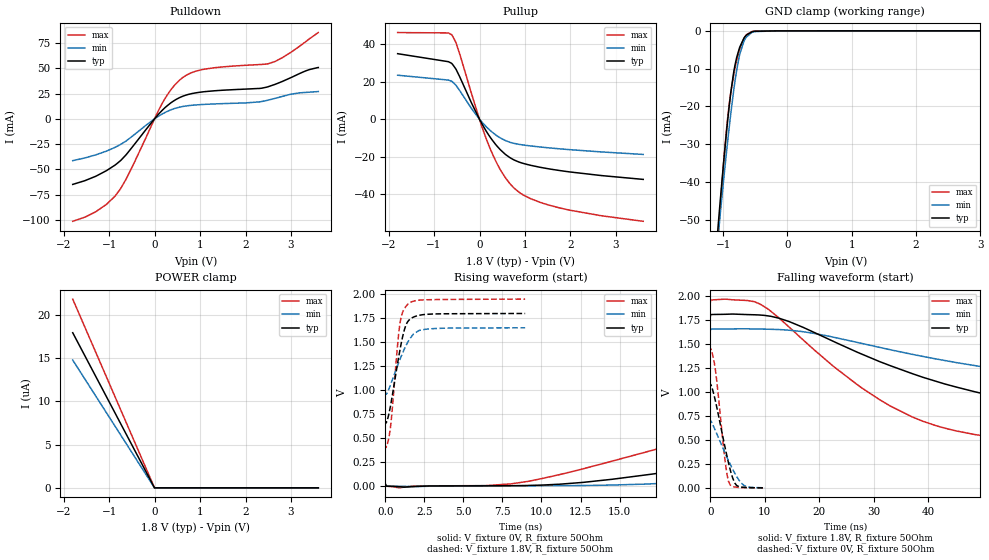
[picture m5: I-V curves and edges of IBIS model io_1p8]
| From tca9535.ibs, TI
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|   io_1p8 Model
[Model]   io_1p8
Model_type   I/O
Polarity   Non-Inverting
Enable   Active-Low
Vinl = 0.54
Vinh = 1.26
Vmeas = 0.9
Vref = 0
Cref = 100pF
Rref = 70
|   typ   min   max
C_comp   2.162e-12   2.013e-12   2.364e-12
[Model spec]
|subparameter
Vinl   0.54   0.495   0.585
Vinh   1.26   1.155   1.365
| Where nom  PVT is Nominal Process, 1.8V, 27C
|   Fast PVT is Strong Process,  1.95V, -40C
|   Slow PVT is Weak Process,   1.65V, 100C
[Voltage Range]   1.8   1.65   1.95
|Junction Temperature
[Temperature Range]   27   100   -40
[Pullup Reference]   1.8   1.65   1.95
[Pulldown Reference]   0   0   0
[Power Clamp Reference]   1.8   1.65   1.95
[GND Clamp Reference]   0   0   0
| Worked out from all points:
|   slope of the pulldown table from 0 to 0.27 V, typ, clamps not added: 21.4 ohm
|   slope of the pullup table from 0 to 0.27 V, typ, clamps not added: 25.1 ohm
|   GND clamp passes 1 mA (typ) near -0.63 V on its own axis
|   falling waveform, V_fixture 1.8V, R_fixture 50Ohm: 20-80 % time 38.2ns typ, 49.8ns min, 23.3ns max; typ from 1.8 V to 0.655 V
|   rising waveform, V_fixture 0V, R_fixture 50Ohm: 20-80 % time 41.8ns typ, 53.4ns min, 26.9ns max; typ from 0 V to 1.07 V
|   rising waveform, V_fixture 1.8V, R_fixture 50Ohm: 20-80 % time 743ps typ, 1.06ns min, 499ps max; typ from 0.653 V to 1.8 V
|   falling waveform, V_fixture 0V, R_fixture 50Ohm: 20-80 % time 2.43ns typ, 3.36ns min, 1.61ns max; typ from 1.07 V to 0.003 V
[Pulldown]
|   Voltage   I(typ)   I(min)   I(max)
-1.8V     -64.95mA   -41.41mA   -101.5mA
-1.288V   -56.76mA   -35.59mA   -91.87mA
-847.9mV  -45.06mA   -27.75mA   -75.37mA
-608.7mV  -34.62mA   -21.35mA   -58.12mA
203.1mV   10.02mA    5.717mA    18.16mA
430.8mV   18.11mA    10.12mA    32.89mA
623.9mV   22.5mA     12.3mA     41.06mA
1.113V    27.02mA    14.39mA    49.37mA
2.317V    30.18mA    16.88mA    53.84mA
2.648V    34.17mA    20.3mA     56.83mA
3.011V    41.15mA    24.57mA    66.34mA
3.6V      50.92mA    27.07mA    85.51mA
[GND Clamp]
|   Voltage   I(typ)   I(min)   I(max)
-1.8V     -224.5mA   -202.8mA   -264.1mA
-1.158V   -68.45mA   -69.08mA   -74.77mA
-1.066V   -49.01mA   -52.08mA   -51.39mA
-1.037V   -43.23mA   -46.97mA   -44.54mA
-990.8mV  -34.41mA   -39.08mA   -34.34mA
-932.3mV  -24.09mA   -29.56mA   -23.33mA
-883.8mV  -16.69mA   -22.24mA   -16.6mA
-837mV    -11.05mA   -15.87mA   -11.74mA
-740.7mV  -4.259mA   -6.106mA   -4.697mA
-665.1mV  -1.66mA    -2.341mA   -1.627mA
-554mV    -267.7uA   -441.4uA   -194.2uA
3.6V      0A         0A         0A
[Pullup]
|   Voltage   I(typ)   I(min)   I(max)
-1.8V     35.04mA    23.52mA    46.35mA
-684mV    30.77mA    20.92mA    46.17mA
-598.8mV  29.53mA    20.05mA    44.75mA
-509.7mV  26.38mA    17.85mA    40.37mA
1.8mV     -167.6uA   -102.1uA   -284.1uA
245.5mV   -10.05mA   -6.293mA   -16.47mA
391.2mV   -14.6mA    -9.037mA   -24.07mA
557.5mV   -18.61mA   -11.32mA   -30.95mA
861.8mV   -22.91mA   -13.45mA   -38.99mA
1.328V    -25.75mA   -14.89mA   -44.5mA
1.76V     -27.5mA    -15.88mA   -47.51mA
3.6V      -32.24mA   -18.88mA   -54.68mA
[POWER Clamp]
|   Voltage   I(typ)   I(min)   I(max)
-1.8V     17.95uA    14.79uA    21.84uA
-54.3mV   524.5nA    435.2nA    636.3nA
-2.1mV    0A         0A         0A
3.6V      0A         0A         0A
[Ramp]
R_load = 50
|   typ   min   max
dV/dt_r   0.641354/4.16014e-08   0.410832/5.32308e-08   0.866703/2.69125e-08
dV/dt_f   0.686979/3.8094e-08   0.415892/4.96413e-08   0.930695/2.32883e-08
[Falling Waveform]
V_fixture = 1.8V
V_fixture_min = 1.65V
V_fixture_max = 1.95V
R_fixture = 50Ohm
|   Time   V(typ)   V(min)   V(max)
0s        1.8V       1.65V      1.95V
9.173ns   1.798V     1.652V     1.912V
14.52ns   1.73V      1.64V      1.671V
23.09ns   1.512V     1.562V     1.244V
32.88ns   1.276V     1.44V      859.9mV
41.37ns   1.112V     1.343V     650.7mV
52.57ns   950.6mV    1.239V     523.8mV
69.05ns   808.3mV    1.131V     451.8mV
93.24ns   717.1mV    1.041V     416.3mV
200ns     655mV      956.8mV    398.8mV
[Rising Waveform]
V_fixture = 0V
V_fixture_min = 0V
V_fixture_max = 0V
R_fixture = 50Ohm
|   Time   V(typ)   V(min)   V(max)
0s        239.1uV    261.6uV    197.6uV
9.173ns   3.748mV    137.6uV    47.16mV
14.52ns   67.89mV    7.953mV    257mV
25.7ns    319.2mV    105.7mV    717.1mV
36.91ns   542.2mV    235.5mV    1.049V
45.22ns   671.2mV    319.9mV    1.204V
56.57ns   802.6mV    413.4mV    1.317V
77.09ns   942.4mV    529.8mV    1.396V
104ns     1.02V      612.3mV    1.429V
200ns     1.069V     685mV      1.445V
[Rising Waveform]
V_fixture = 1.8V
V_fixture_min = 1.65V
V_fixture_max = 1.95V
R_fixture = 50Ohm
|   Time   V(typ)   V(min)   V(max)
0s        653mV      952.8mV    398.6mV
176.2ps   716.7mV    990.7mV    466.6mV
341ps     845mV      1.059V     631.2mV
775ps     1.27V      1.251V     1.457V
931.8ps   1.415V     1.317V     1.69V
1.108ns   1.557V     1.387V     1.811V
1.399ns   1.704V     1.487V     1.888V
1.805ns   1.76V      1.585V     1.926V
2.559ns   1.788V     1.633V     1.941V
8.953ns   1.798V     1.648V     1.948V
[Falling Waveform]
V_fixture = 0V
V_fixture_min = 0V
V_fixture_max = 0V
R_fixture = 50Ohm
|   Time   V(typ)   V(min)   V(max)
0s        1.072V     691.1mV    1.445V
447.9ps   1.017V     660.2mV    1.38V
957.8ps   900.6mV    595.1mV    1.22V
2.559ns   464.4mV    384.7mV    361.7mV
3.003ns   347.8mV    328.3mV    167.5mV
3.349ns   262.6mV    285.5mV    70.47mV
4.108ns   106.3mV    196.5mV    17.61mV
4.834ns   27.5mV     121.3mV    9.4mV
6.816ns   6.151mV    12.51mV    3.949mV
9.986ns   2.741mV    3.546mV    2.703mV
